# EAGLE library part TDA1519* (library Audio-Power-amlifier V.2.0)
22WBTL or 2 ´ 11Wstereo power amplifier
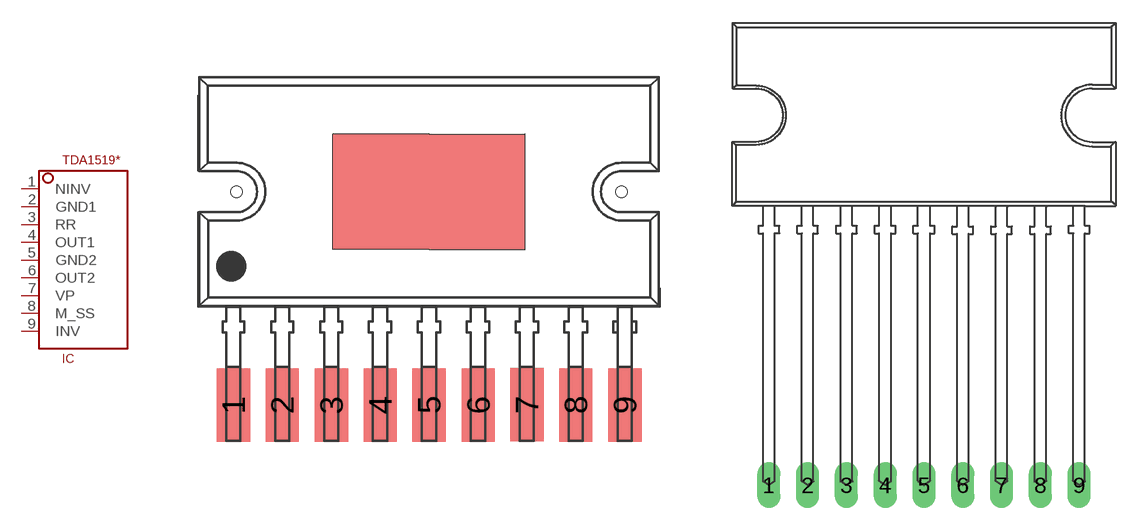
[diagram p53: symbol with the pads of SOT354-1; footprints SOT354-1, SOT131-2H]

Designator prefix IC

## TDA1519TDA1519CSP  [SOT354-1]
1  NINV
2  GND1  pwr
3  RR
4  OUT1  out
5  GND2  pwr
6  OUT2  out
7  VP  pwr
8  M_SS
9  INV

## TDA1519TDA1519C  [SOT131-2H]
Pads as for SOT354-1

## TDA1519TDA1519  [SOT110-1]
Pads as for SOT354-1

## TDA1519TDA1519A  [SOT157-2]
Pads as for SOT354-1

## Footprint SOT354-1 (pad centres in mm)
smd 1.73 x 3.81: 1 -10.15,-5.1; 2 -7.62,-5.09; 3 -5.07,-5.1; 4 -2.53,-5.09; 5 0,-5.09; 6 2.56,-5.09; 7 5.08,-5.08; 8 7.62,-5.09; 9 10.17,-5.09
hole 0.6 at -10,6
hole 0.6 at 10,6

## Footprint SOT131-2H (pad centres in mm)
drill 1 long: 1 -10.16,0; 2 -7.62,0; 3 -5.08,0; 4 -2.54,0; 5 0,0; 6 2.54,0; 7 5.08,0; 8 7.62,0; 9 10.16,0

## Footprint SOT110-1 (pad centres in mm)
SIL9MPF: plastic single in-line medium power package with fin; 9 leads
drill 0.8 long: 1 -10.16,0; 2 -7.62,0; 3 -5.08,0; 4 -2.54,0; 5 0,0; 6 2.54,0; 7 5.08,0; 8 7.62,0; 9 10.16,0

## Footprint SOT157-2 (pad centres in mm)
drill 1 long: 1 -10.16,0; 2 -7.62,-2.54; 3 -5.08,0; 4 -2.54,-2.54; 5 0,0; 6 2.54,-2.54; 7 5.08,0; 8 7.62,-2.54; 9 10.16,0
